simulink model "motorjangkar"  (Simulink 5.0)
settings: Solver=ode45  StartTime=0.0  StopTime=6  RelTol=1e-3
libraries: simulink x1

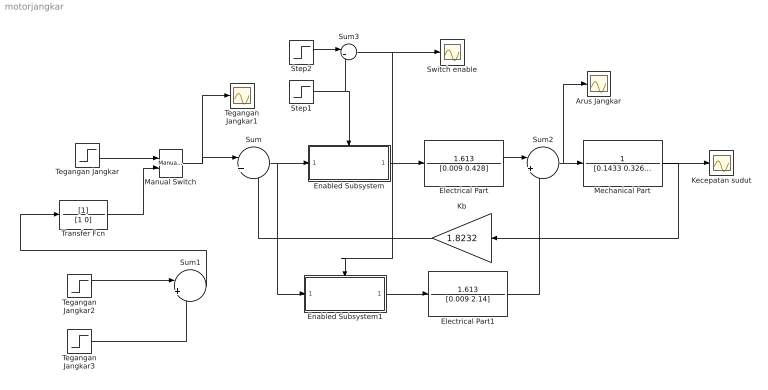
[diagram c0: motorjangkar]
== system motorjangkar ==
  Arus Jangkar : Scope
  Electrical Part : TransferFcn  Numerator=1.613  Denominator=[0.009 0.428]
  Electrical Part1 : TransferFcn  Numerator=1.613  Denominator=[0.009 2.14]
  Enabled Subsystem : Subsystem  TreatAsAtomicUnit=on
  Enabled Subsystem1 : Subsystem  TreatAsAtomicUnit=on
  Kb : Gain  Orientation=left  Gain=1.8232
  Kecepatan sudut : Scope
  Manual Switch : simulink/Signal Routing/Manual Switch  sw=1  action=0
  Mechanical Part : TransferFcn  Numerator=1  Denominator=[0.1433 0.3265]
  Step1 : Step  Time=5.1  SampleTime=0
  Step2 : Step  Time=0  SampleTime=0
  Sum : Sum  Inputs=|+-
  Sum1 : Sum  Inputs=|+-
  Sum2 : Sum  Inputs=|++
  Sum3 : Sum  Inputs=|+-
  Switch enable : Scope
  Tegangan Jangkar : Step  Time=0.1  After=500  SampleTime=0
  Tegangan Jangkar1 : Scope
  Tegangan Jangkar2 : Step  Time=0.1  After=25  SampleTime=0
  Tegangan Jangkar3 : Step  Time=20.1  After=25  SampleTime=0
  Transfer Fcn : TransferFcn  Denominator=[1 0]
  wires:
  Kb/1 -> Sum/2
  Mechanical Part/1 -> Kecepatan sudut/1, Kb/1
  Tegangan Jangkar/1 -> Manual Switch/1
  Manual Switch/1 -> Sum/1, Tegangan Jangkar1/1
  Transfer Fcn/1 -> Manual Switch/2
  Tegangan Jangkar2/1 -> Sum1/1
  Tegangan Jangkar3/1 -> Sum1/2
  Sum1/1 -> Transfer Fcn/1
  Sum/1 -> Enabled Subsystem/1(In1), Enabled Subsystem1/1(In1)
  Enabled Subsystem/1(Out1) -> Electrical Part/1
  Electrical Part/1 -> Sum2/1
  Electrical Part1/1 -> Sum2/2
  Sum2/1 -> Mechanical Part/1, Arus Jangkar/1
  Enabled Subsystem1/1(Out1) -> Electrical Part1/1
  Step2/1 -> Sum3/1
  Step1/1 -> Sum3/2, Enabled Subsystem/Enable
  Sum3/1 -> Enabled Subsystem1/Enable, Switch enable/1

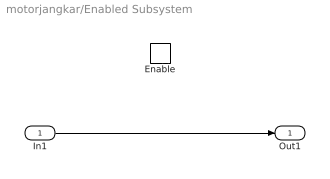
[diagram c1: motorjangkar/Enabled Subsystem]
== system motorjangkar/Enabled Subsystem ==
  In1 : Inport
  Enable : EnablePort
  Out1 : Outport  OutputWhenDisabled=reset  InitialOutput=[0]
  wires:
  In1/1 -> Out1/1

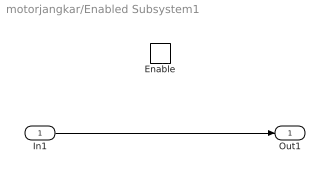
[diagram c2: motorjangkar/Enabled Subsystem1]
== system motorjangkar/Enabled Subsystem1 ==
  In1 : Inport
  Enable : EnablePort
  Out1 : Outport  InitialOutput=[0]
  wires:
  In1/1 -> Out1/1
